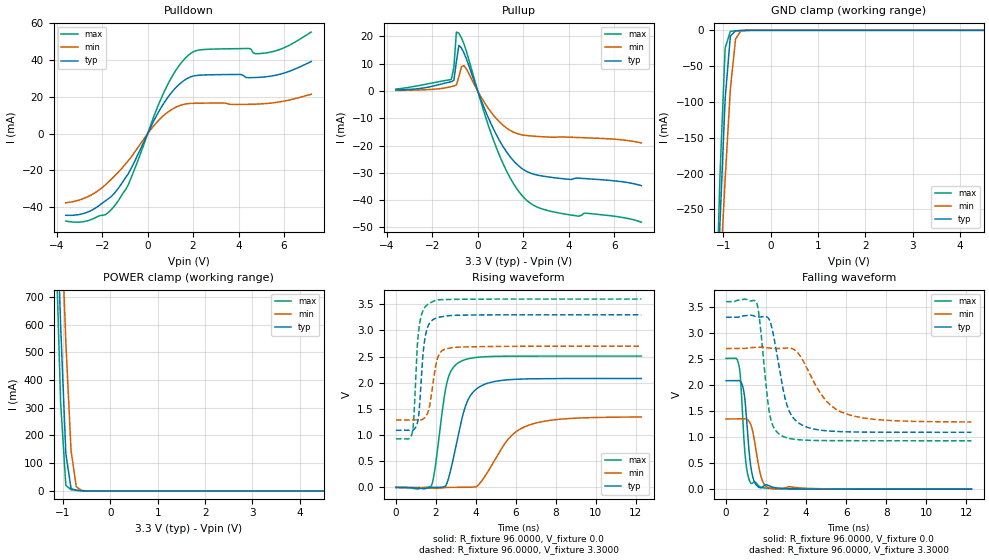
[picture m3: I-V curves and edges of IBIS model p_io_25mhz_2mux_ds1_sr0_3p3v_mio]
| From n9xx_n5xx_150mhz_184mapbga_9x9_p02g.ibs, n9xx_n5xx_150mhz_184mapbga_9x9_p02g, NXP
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[Model] p_io_25mhz_2mux_ds1_sr0_3p3v_mio
|   Model p_io_25mhz_2mux_ds1_sr0_3p3v_mio
| This model was characterised for following simulation conditions:
| External (pad) voltage:
|   - Typ: 3.3V,   - Min: 2.7V,   - Max: 3.6V
| Library cells for typ/min/max conditions are connected as defined below:
|  pad - External Pad
|  ipp_do_lv - Core Input
|  ipp_obe_lv - Output Buffer Enable
|  IOGC - NC
|  REFH3V3 - REFH3V3
|  REFL3V3 - REFL3V3
|  ZI - NC
|  abut_ncal_vddio[1] - vddio
|  abut_ncal_vddio[2] - vddio
|  abut_ncal_vddio[3] - vssio
|  abut_ncal_vddio[4] - vddio
|  abut_ncal_vddio[5] - vddio
|  abut_ncal_vddio[6] - vssio
|  abut_pcal_vddio[1] - vssio
|  abut_pcal_vddio[2] - vssio
|  abut_pcal_vddio[3] - vddio
|  abut_pcal_vddio[4] - vssio
|  abut_pcal_vddio[5] - vssio
|  abut_pcal_vddio[6] - vddio
|  ipp_do_1p8v - ipp_do_1p8v
|  ipp_dse_lv - vdd_lv
|  ipp_eftd_lv - NC
|  ipp_ina_mux_vddio - NC
|  ipp_ina_mux_vddio[0] - NC
|  ipp_ina_mux_vddio[1] - NC
|  ipp_ina_r0_vddio - NC
|  ipp_ina_r0a_vddio - NC
|  ipp_ina_r0b_vddio - NC
|  ipp_ina_r0c_vddio - NC
|  ipp_ina_r0d_vddio - NC
|  ipp_ina_r0e_vddio - NC
|  ipp_ina_r0f_vddio - NC
|  ipp_ina_r300_vddio - NC
|  ipp_ina_r300a_vddio - NC
|  ipp_ina_r300b_vddio - NC
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Model_type I/O
Polarity   Non-Inverting
Enable   Active-High
Vinl =   0.9900V
Vinh =   2.3100V
Vmeas =  1.6500V
Cref =   30.0000pF
Rref =   1.0000M
Vref =   3.3000V
C_comp   1.2811pF   1.2303pF   1.3501pF
|C_comp_pullup   0.5366pF   0.5677pF   0.5153pF
|C_comp_pulldown   0.6709pF   0.7076pF   0.6417pF
[Model Spec]
| variable   typ   min   max
Vinh   2.3100V   1.8900V   2.5200V
Vinl   0.9900V   0.8100V   1.0800V
[Temperature Range]   25.0000   0.1250k   -40.0000
[Voltage Range]   3.3000V   2.7000V   3.6000V
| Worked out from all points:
|   slope of the pulldown table from 0 to 0.495 V, typ, clamps not added: 40.8 ohm
|   slope of the pullup table from 0 to 0.495 V, typ, clamps not added: 47.8 ohm
|   GND clamp passes 1 mA (typ) near -0.74 V on its own axis
|   POWER clamp passes 1 mA (typ) near -0.62 V on its own axis
|   rising waveform, R_fixture 96.0000, V_fixture 0.0: 20-80 % time 805ps typ, 1.51ns min, 548ps max; typ from 0 V to 2.08 V
|   rising waveform, R_fixture 96.0000, V_fixture 3.3000: 20-80 % time 277ps typ, 351ps min, 247ps max; typ from 1.09 V to 3.3 V
|   falling waveform, R_fixture 96.0000, V_fixture 0.0: 20-80 % time 287ps typ, 380ps min, 249ps max; typ from 2.08 V to 0 V
|   falling waveform, R_fixture 96.0000, V_fixture 3.3000: 20-80 % time 698ps typ, 1.44ns min, 438ps max; typ from 3.3 V to 1.09 V
[Pulldown]
|Voltage   I(typ)   I(min)   I(max)
-3.6V     -44.37mA   -37.58mA   -47.51mA
-2.5V     -41.88mA   -33.45mA   -46.76mA
-1.84V    -36.35mA   -27.58mA   -43.92mA
-1.4V     -31.43mA   -22.29mA   -38.34mA
-850mV    -21.79mA   -14.63mA   -27.74mA
800mV     18.21mA    10.89mA    24.66mA
1.35V     26.41mA    15.03mA    36.45mA
1.9V      30.96mA    16.49mA    43.73mA
4.43V     30.52mA    16mA       46.39mA
4.76V     30.6mA     16.11mA    43.53mA
5.31V     31.15mA    16.53mA    44.19mA
7.2V      39.28mA    21.46mA    55.3mA
[Pullup]
|Voltage   I(typ)   I(min)   I(max)
-3.6V     375uA      207.1uA    721uA
-1.16V    3.419mA    1.608mA    4.218mA
-1.05V    3.929mA    1.825mA    8.684mA
-940mV    10.66mA    2.209mA    21.58mA
-830mV    16.7mA     5.227mA    21.23mA
-720mV    15.82mA    8.86mA     19.48mA
-610mV    14mA       9.299mA    17.3mA
820mV     -16.02mA   -10.13mA   -20.76mA
1.48V     -24.66mA   -14.68mA   -32.62mA
2.03V     -28.88mA   -16.19mA   -39.03mA
3.35V     -31.76mA   -16.97mA   -44.31mA
7.2V      -34.67mA   -19.04mA   -48.06mA
[GND_clamp]
|Voltage   I(typ)   I(min)   I(max)
-3.6V     -5.309A    -4.128A    -6.876A
-1.18V    -466mA     -495.4mA   -458.9mA
-1.07V    -271.1mA   -348.5mA   -204.6mA
-960mV    -95.65mA   -208mA     -24.74mA
-850mV    -8.096mA   -81.85mA   -1.471mA
-740mV    -719.7uA   -12.14mA   -717.6uA
-630mV    -272.5uA   -923.5uA   -300.8uA
-300mV    -385.6nA   -2.502uA   -74.88nA
7.2V      0A         0A         0A
[POWER_clamp]
|Voltage   I(typ)   I(min)   I(max)
-3.6V     14.48A     12.95A     16.35A
-1.16V    1.177A     1.535A     951.2mA
-1.05V    598.4mA    1.032A     318mA
-940mV    134.2mA    537.3mA    20.02mA
-830mV    8.708mA    145.4mA    4.242mA
-720mV    2.127mA    15.38mA    2.218mA
-610mV    847.4uA    1.853mA    834.1uA
7.2V      0A         0A         0A
[Ramp]
| variable   typ   min   max
dV/dt_r  1.2493/0.8052n   0.8077/1.5056n   1.5061/0.5479n
dV/dt_f  1.3249/0.6980n   0.8455/1.4379n   1.6024/0.4383n
R_load = 96.0000
[Rising Waveform]
R_fixture= 96.0000
V_fixture= 0.0
V_fixture_min= 0.0
V_fixture_max= 0.0
|time   V(typ)   V(min)   V(max)
0s        3.081nV    103.2nV    10.53nV
1.779ns   353.8uV    -13.83mV   35.85mV
1.96ns    1.977mV    -17.2mV    379mV
2.532ns   63.09mV    -76.98uV   1.974V
3.2ns     1.15V      1.285mV    2.401V
3.715ns   1.75V      2.486mV    2.467V
4.695ns   2.004V     363mV      2.502V
5.663ns   2.059V     945mV      2.509V
6.664ns   2.076V     1.193V     2.51V
12.27ns   2.082V     1.346V     2.51V
[Rising Waveform]
R_fixture= 96.0000
V_fixture= 3.3000
V_fixture_min= 2.7000
V_fixture_max= 3.6000
|time   V(typ)   V(min)   V(max)
0s        1.092V     1.289V     929.3mV
813.4ps   1.091V     1.289V     1.039V
900.3ps   1.107V     1.289V     1.361V
1.064ns   1.22V      1.289V     2.684V
1.165ns   1.481V     1.288V     3.078V
1.396ns   2.7V       1.317V     3.412V
1.659ns   3.124V     1.51V      3.515V
2.057ns   3.243V     2.438V     3.581V
2.505ns   3.274V     2.648V     3.592V
12.27ns   3.3V       2.7V       3.6V
[Falling Waveform]
R_fixture= 96.0000
V_fixture= 0.0
V_fixture_min= 0.0
V_fixture_max= 0.0
|time   V(typ)   V(min)   V(max)
0s        2.082V     1.348V     2.51V
644.6ps   2.085V     1.348V     2.375V
732.2ps   2.063V     1.348V     2.08V
871.9ps   1.911V     1.35V      1.091V
971.7ps   1.605V     1.35V      579.7mV
1.256ns   387.5mV    1.218V     111.2mV
1.443ns   121.5mV    880.2mV    138mV
1.752ns   27.46mV    238.5mV    36.05mV
2.176ns   58.84mV    20.97mV    15mV
12.27ns   224.4nV    15.75uV    31.24nV
[Falling Waveform]
R_fixture= 96.0000
V_fixture= 3.3000
V_fixture_min= 2.7000
V_fixture_max= 3.6000
|time   V(typ)   V(min)   V(max)
0s        3.3V       2.7V       3.6V
1.531ns   3.312V     2.723V     3.577V
1.683ns   3.304V     2.727V     3.235V
2.173ns   3.247V     2.707V     1.456V
2.758ns   2.104V     2.703V     1.031V
3.255ns   1.426V     2.701V     966.9mV
4.168ns   1.175V     2.227V     937.9mV
5.035ns   1.12V      1.684V     932mV
6.17ns    1.1V       1.425V     930mV
12.27ns   1.092V     1.291V     929.3mV
